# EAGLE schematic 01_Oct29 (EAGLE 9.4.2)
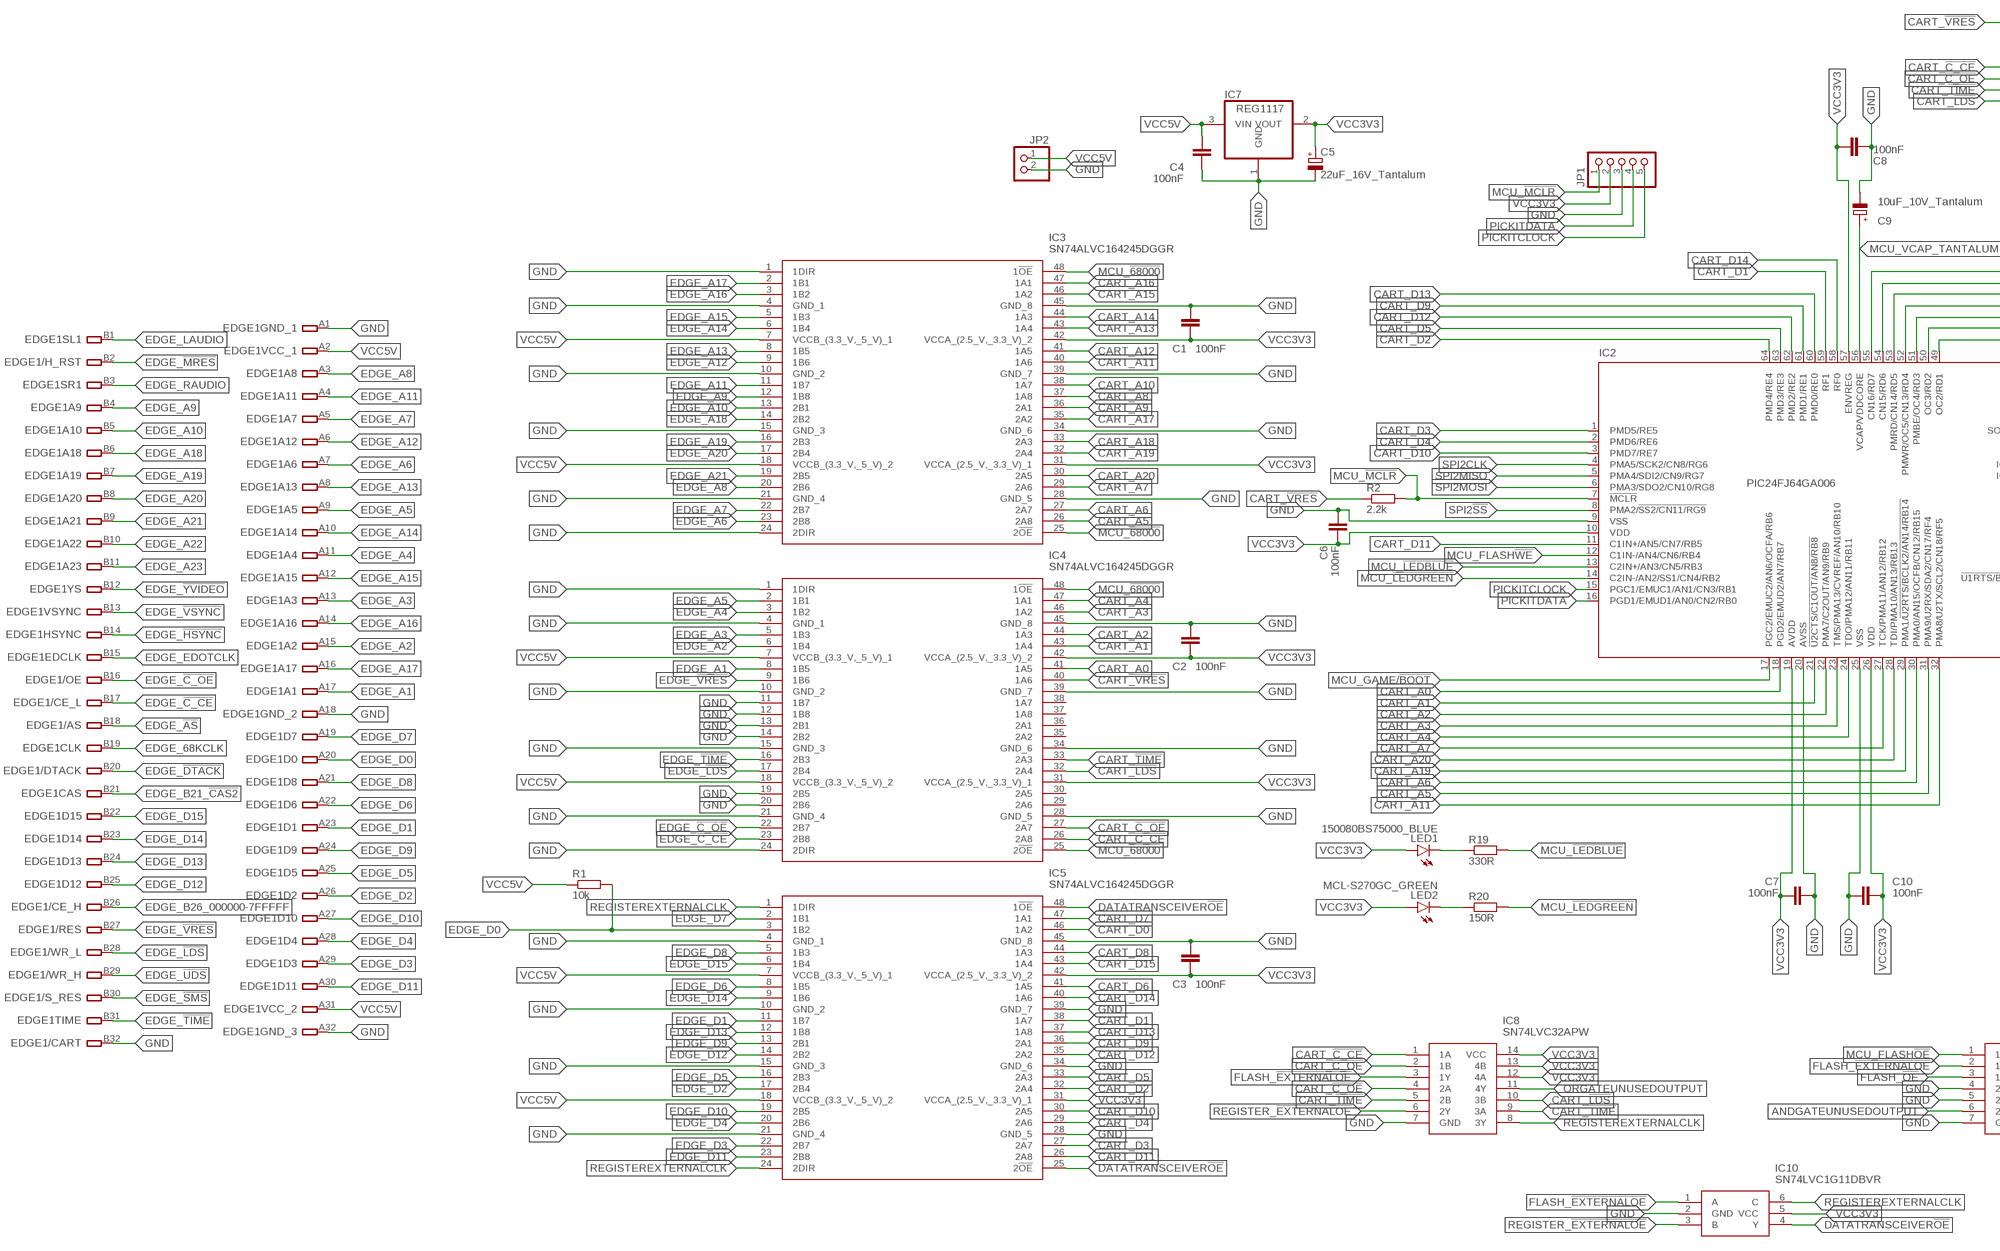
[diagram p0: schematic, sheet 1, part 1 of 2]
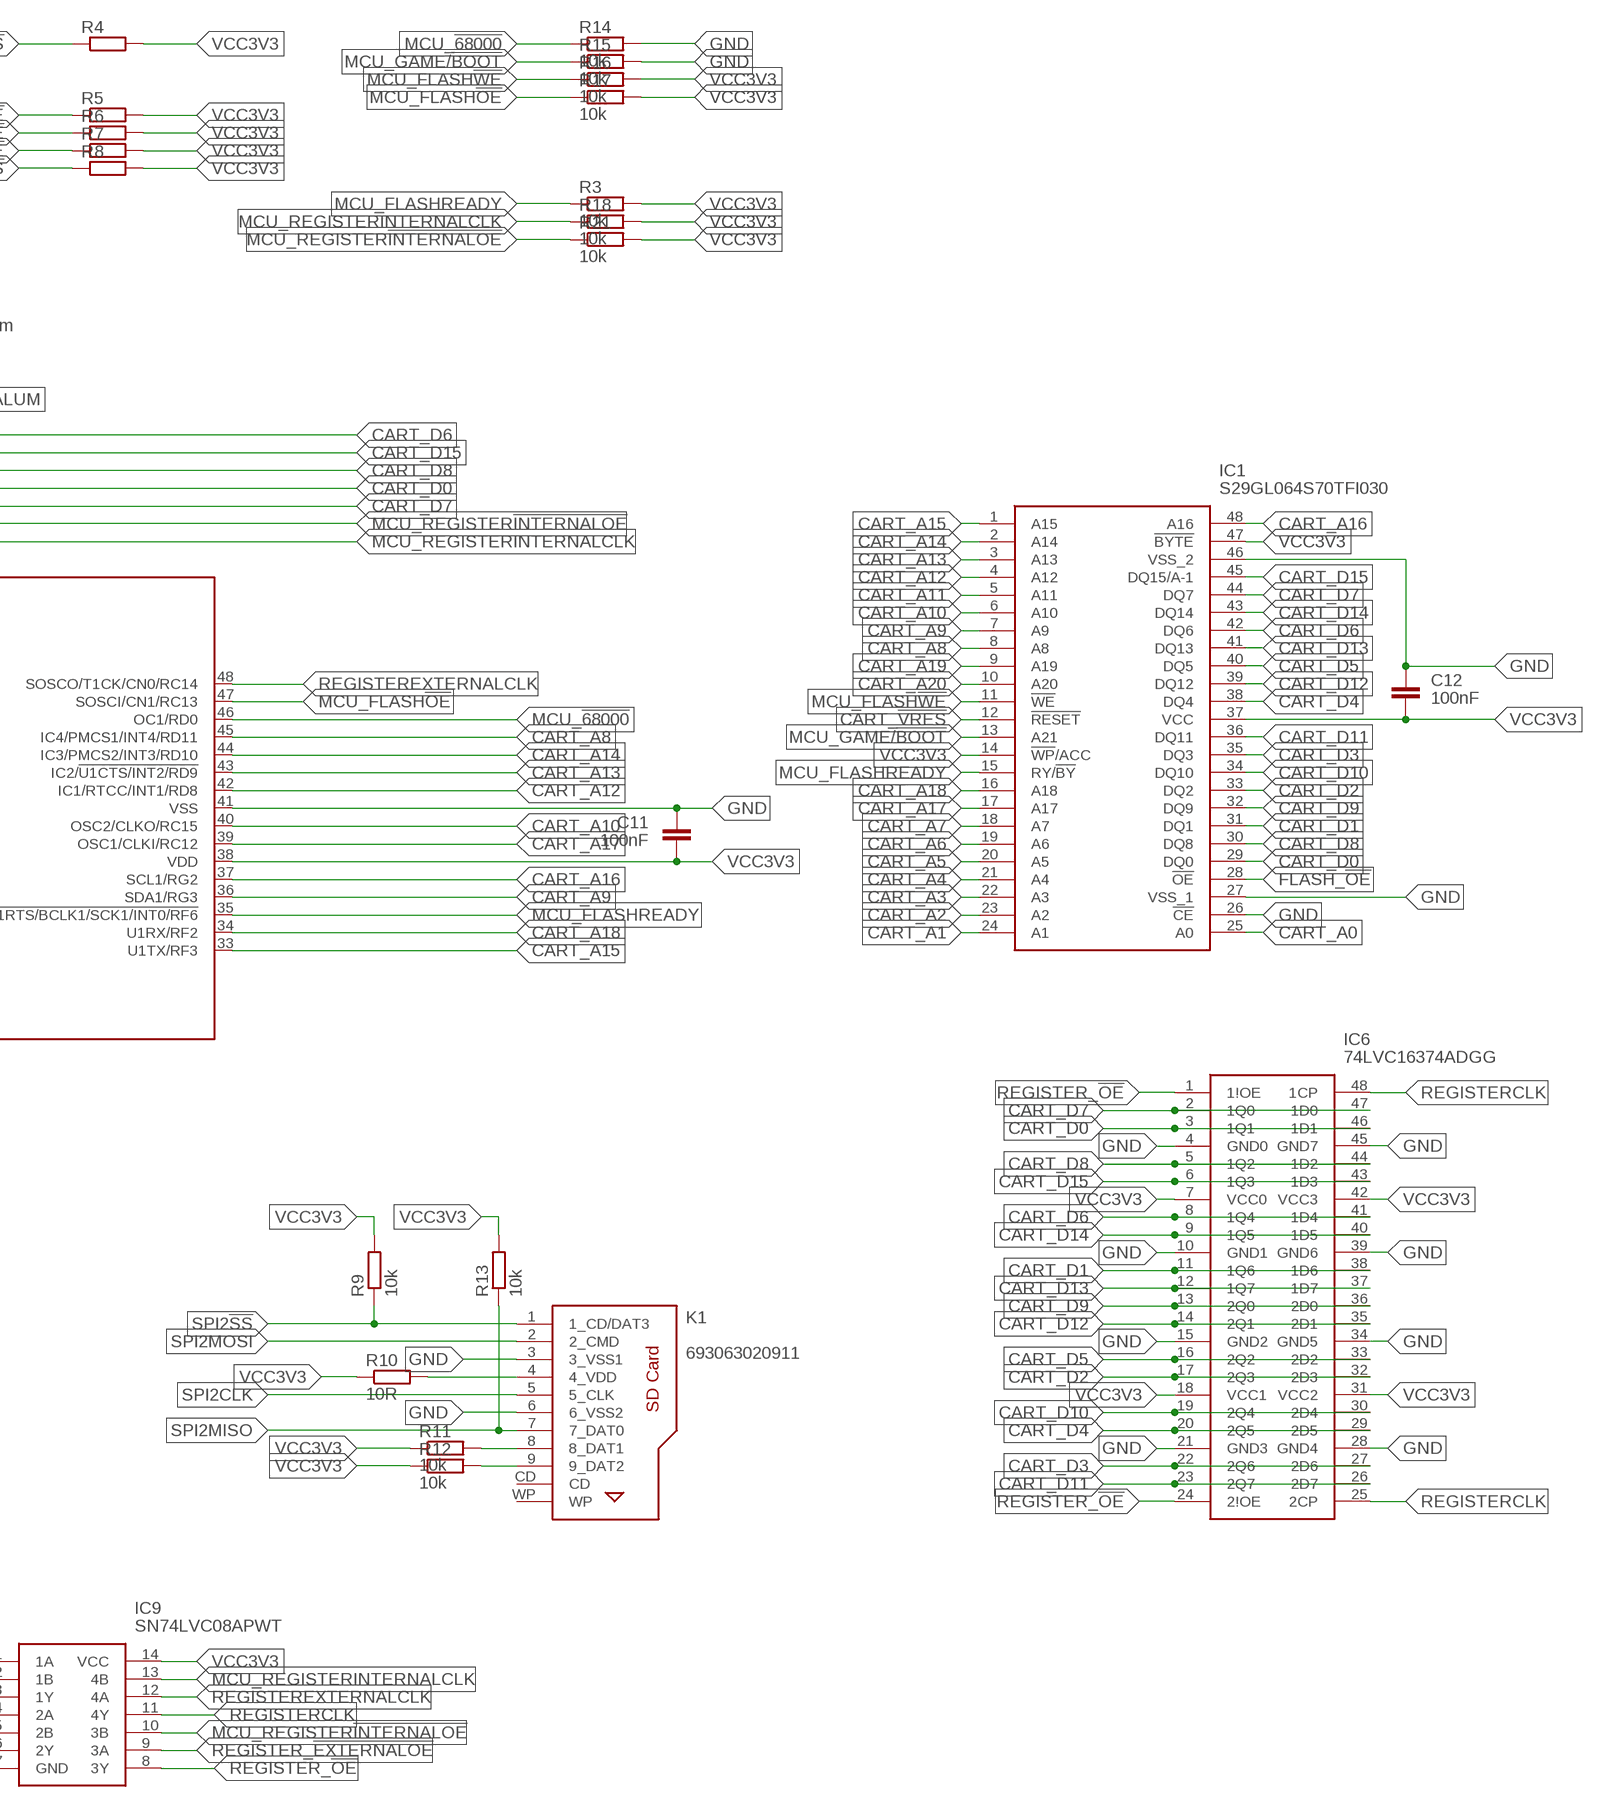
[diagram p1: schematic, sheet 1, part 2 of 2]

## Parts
C1  100nF  C-EUC0603  [C0603]
C2  100nF  C-EUC0603  [C0603]
C3  100nF  C-EUC0603  [C0603]
C4  100nF  C-EUC0603  [C0603]
C5  22uF_16V_Tantalum  CPOL-EUCT3528  [CT3528]
C6  100nF  C-EUC0603  [C0603]
C7  100nF  C-EUC0603  [C0603]
C8  100nF  C-EUC0603  [C0603]
C9  10uF_10V_Tantalum  CPOL-EUCT3216  [CT3216]
C10  100nF  C-EUC0603  [C0603]
C11  100nF  C-EUC0603  [C0603]
C12  100nF  C-EUC0603  [C0603]
EDGE1  GENESIS-LARGE  [GENESIS-LARGE]
IC1  S29GL064S70TFI030  [SOP50P2000X120-48N]
IC2  PIC24FJ64GA006  [TQFP64-10X10]
IC3  SN74ALVC164245DGGR  [SOP50P810X120-48N]
IC4  SN74ALVC164245DGGR  [SOP50P810X120-48N]
IC5  SN74ALVC164245DGGR  [SOP50P810X120-48N]
IC6  74LVC16374ADGG  [SOP50P810X120-48N]
IC7  REG1117  [SOT223]
IC8  SN74LVC32APW  [SOP65P640X120-14N]
IC9  SN74LVC08APWT  [SOP65P640X120-14N]
IC10  SN74LVC1G11DBVR  [SOT95P280X145-6N]
JP1  PINHD-1X5  [1X05]
JP2  PINHD-1X2  [1X02]
K1  693063020911  [693063020911]
LED1  150080BS75000_BLUE  LEDSML0805  [SML0805]
LED2  MCL-S270GC_GREEN  LEDSML0805  [SML0805]
R1  10k  R-EU_R0402  [R0402]
R2  2.2k  R-EU_R0402  [R0402]
R3  10k  R-EU_R0402  [R0402]
R4  10k  R-EU_R0402  [R0402]
R5  10k  R-EU_R0402  [R0402]
R6  10k  R-EU_R0402  [R0402]
R7  10k  R-EU_R0402  [R0402]
R8  10k  R-EU_R0402  [R0402]
R9  10k  R-EU_R0402  [R0402]
R10  10R  R-EU_R0402  [R0402]
R11  10k  R-EU_R0402  [R0402]
R12  10k  R-EU_R0402  [R0402]
R13  10k  R-EU_R0402  [R0402]
R14  10k  R-EU_R0402  [R0402]
R15  10k  R-EU_R0402  [R0402]
R16  10k  R-EU_R0402  [R0402]
R17  10k  R-EU_R0402  [R0402]
R18  10k  R-EU_R0402  [R0402]
R19  330R  R-EU_R0402  [R0402]
R20  150R  R-EU_R0402  [R0402]
R21  10k  R-EU_R0402  [R0402]

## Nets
ANDGATEUNUSEDOUTPUT: IC9.6(2Y)
CART_!C_CE: IC4.26(2A8) IC8.1(1A) R5.1
CART_!C_OE: IC4.27(2A7) IC8.2(1B) IC8.4(2A) R6.1
CART_!LDS: IC4.32(2A4) IC8.10(3B) R8.1
CART_!TIME: IC4.33(2A3) IC8.5(2B) IC8.9(3A) R7.1
CART_!VRES: IC1.12(!RESET) IC4.40(1A6) R2.1 R4.1
CART_A0: IC1.25(A0) IC2.18(PGD2/EMUD2/AN7/RB7) IC4.41(1A5)
CART_A1: IC1.24(A1) IC2.21(!U2CTS/C1OUT/AN8/RB8) IC4.43(1A4)
CART_A2: IC1.23(A2) IC2.22(PMA7/C2OUT/AN9/RB9) IC4.44(1A3)
CART_A3: IC1.22(A3) IC2.23(TMS/PMA13/CVREF/AN10/RB10) IC4.46(1A2)
CART_A4: IC1.21(A4) IC2.24(TDO/PMA12/AN11/RB11) IC4.47(1A1)
CART_A5: IC1.20(A5) IC2.31(PMA9/U2RX/SDA2/CN17/RF4) IC3.26(2A8)
CART_A6: IC1.19(A6) IC2.30(PMA0/AN15/OCFB/CN12/RB15) IC3.27(2A7)
CART_A7: IC1.18(A7) IC2.27(TCK/PMA11/AN12/RB12) IC3.29(2A6)
CART_A8: IC1.8(A8) IC2.45(IC4/PMCS1/INT4/RD11) IC3.37(1A8)
CART_A9: IC1.7(A9) IC2.36(SDA1/RG3) IC3.36(2A1)
CART_A10: IC1.6(A10) IC2.40(OSC2/CLKO/RC15) IC3.38(1A7)
CART_A11: IC1.5(A11) IC2.32(PMA8/U2TX/SCL2/CN18/RF5) IC3.40(1A6)
CART_A12: IC1.4(A12) IC2.42(IC1/RTCC/INT1/RD8) IC3.41(1A5)
CART_A13: IC1.3(A13) IC2.43(IC2/!U1CTS/INT2/RD9) IC3.43(1A4)
CART_A14: IC1.2(A14) IC2.44(IC3/PMCS2/INT3/RD10) IC3.44(1A3)
CART_A15: IC1.1(A15) IC2.33(U1TX/RF3) IC3.46(1A2)
CART_A16: IC1.48(A16) IC2.37(SCL1/RG2) IC3.47(1A1)
CART_A17: IC1.17(A17) IC2.39(OSC1/CLKI/RC12) IC3.35(2A2)
CART_A18: IC1.16(A18) IC2.34(U1RX/RF2) IC3.33(2A3)
CART_A19: IC1.9(A19) IC2.29(PMA1/!U2RTS/BCLK2/AN14/RB14) IC3.32(2A4)
CART_A20: IC1.10(A20) IC2.28(TDI/PMA10/AN13/RB13) IC3.30(2A5)
CART_D0: IC1.29(DQ0) IC2.52(PMWR/OC5/CN13/RD4) IC5.46(1A2) IC6.3(1Q1) IC6.46(1D1)
CART_D1: IC1.31(DQ1) IC2.59(RF1) IC5.38(1A7) IC6.11(1Q6) IC6.38(1D6)
CART_D2: IC1.33(DQ2) IC2.64(PMD4/RE4) IC5.32(2A4) IC6.17(2Q3) IC6.32(2D3)
CART_D3: IC1.35(DQ3) IC2.1(PMD5/RE5) IC5.27(2A7) IC6.22(2Q6) IC6.27(2D6)
CART_D4: IC1.38(DQ4) IC2.2(PMD6/RE6) IC5.29(2A6) IC6.20(2Q5) IC6.29(2D5)
CART_D5: IC1.40(DQ5) IC2.63(PMD3/RE3) IC5.33(2A3) IC6.16(2Q2) IC6.33(2D2)
CART_D6: IC1.42(DQ6) IC2.55(CN16/RD7) IC5.41(1A5) IC6.8(1Q4) IC6.41(1D4)
CART_D7: IC1.44(DQ7) IC2.51(PMBE/OC4/RD3) IC5.47(1A1) IC6.2(1Q0) IC6.47(1D0)
CART_D8: IC1.30(DQ8) IC2.53(PMRD/CN14/RD5) IC5.44(1A3) IC6.5(1Q2) IC6.44(1D2)
CART_D9: IC1.32(DQ9) IC2.61(PMD1/RE1) IC5.36(2A1) IC6.13(2Q0) IC6.36(2D0)
CART_D10: IC1.34(DQ10) IC2.3(PMD7/RE7) IC5.30(2A5) IC6.19(2Q4) IC6.30(2D4)
CART_D11: IC1.36(DQ11) IC2.11(C1IN+/AN5/CN7/RB5) IC5.26(2A8) IC6.23(2Q7) IC6.26(2D7)
CART_D12: IC1.39(DQ12) IC2.62(PMD2/RE2) IC5.35(2A2) IC6.14(2Q1) IC6.35(2D1)
CART_D13: IC1.41(DQ13) IC2.60(PMD0/RE0) IC5.37(1A8) IC6.12(1Q7) IC6.37(1D7)
CART_D14: IC1.43(DQ14) IC2.58(RF0) IC5.40(1A6) IC6.9(1Q5) IC6.40(1D5)
CART_D15: IC1.45(DQ15/A-1) IC2.54(CN15/RD6) IC5.43(1A4) IC6.6(1Q3) IC6.43(1D3)
DATATRANSCEIVER!OE: IC5.25(2!OE) IC5.48(1!OE) IC10.4(Y)
EDGE_68KCLK: EDGE1.B19
EDGE_!AS: EDGE1.B18
EDGE_!C_CE: EDGE1.B17 IC4.23(2B8)
EDGE_!C_OE: EDGE1.B16 IC4.22(2B7)
EDGE_!DTACK: EDGE1.B20
EDGE_!HSYNC: EDGE1.B14
EDGE_!LDS: EDGE1.B28 IC4.17(2B4)
EDGE_!MRES: EDGE1.B2
EDGE_!SMS: EDGE1.B30
EDGE_!TIME: EDGE1.B31 IC4.16(2B3)
EDGE_!UDS: EDGE1.B29
EDGE_!VRES: EDGE1.B27 IC4.9(1B6)
EDGE_!VSYNC: EDGE1.B13
EDGE_!YVIDEO: EDGE1.B12
EDGE_A1: EDGE1.A17 IC4.8(1B5)
EDGE_A2: EDGE1.A15 IC4.6(1B4)
EDGE_A3: EDGE1.A13 IC4.5(1B3)
EDGE_A4: EDGE1.A11 IC4.3(1B2)
EDGE_A5: EDGE1.A9 IC4.2(1B1)
EDGE_A6: EDGE1.A7 IC3.23(2B8)
EDGE_A7: EDGE1.A5 IC3.22(2B7)
EDGE_A8: EDGE1.A3 IC3.20(2B6)
EDGE_A9: EDGE1.B4 IC3.12(1B8)
EDGE_A10: EDGE1.B5 IC3.13(2B1)
EDGE_A11: EDGE1.A4 IC3.11(1B7)
EDGE_A12: EDGE1.A6 IC3.9(1B6)
EDGE_A13: EDGE1.A8 IC3.8(1B5)
EDGE_A14: EDGE1.A10 IC3.6(1B4)
EDGE_A15: EDGE1.A12 IC3.5(1B3)
EDGE_A16: EDGE1.A14 IC3.3(1B2)
EDGE_A17: EDGE1.A16 IC3.2(1B1)
EDGE_A18: EDGE1.B6 IC3.14(2B2)
EDGE_A19: EDGE1.B7 IC3.16(2B3)
EDGE_A20: EDGE1.B8 IC3.17(2B4)
EDGE_A21: EDGE1.B9 IC3.19(2B5)
EDGE_A22: EDGE1.B10
EDGE_A23: EDGE1.B11
EDGE_B21_!CAS2: EDGE1.B21
EDGE_B26_000000-7FFFFF: EDGE1.B26
EDGE_D0: EDGE1.A20 IC5.3(1B2) R1.2
EDGE_D1: EDGE1.A23 IC5.11(1B7)
EDGE_D2: EDGE1.A26 IC5.17(2B4)
EDGE_D3: EDGE1.A29 IC5.22(2B7)
EDGE_D4: EDGE1.A28 IC5.20(2B6)
EDGE_D5: EDGE1.A25 IC5.16(2B3)
EDGE_D6: EDGE1.A22 IC5.8(1B5)
EDGE_D7: EDGE1.A19 IC5.2(1B1)
EDGE_D8: EDGE1.A21 IC5.5(1B3)
EDGE_D9: EDGE1.A24 IC5.13(2B1)
EDGE_D10: EDGE1.A27 IC5.19(2B5)
EDGE_D11: EDGE1.A30 IC5.23(2B8)
EDGE_D12: EDGE1.B25 IC5.14(2B2)
EDGE_D13: EDGE1.B24 IC5.12(1B8)
EDGE_D14: EDGE1.B23 IC5.9(1B6)
EDGE_D15: EDGE1.B22 IC5.6(1B4)
EDGE_EDOTCLK: EDGE1.B15
EDGE_LAUDIO: EDGE1.B1
EDGE_RAUDIO: EDGE1.B3
FLASH_!EXTERNALOE: IC8.3(1Y) IC9.2(1B) IC10.1(A)
FLASH_!OE: IC1.28(!OE) IC9.3(1Y)
GND [pow]: C1.2 C2.2 C3.2 C4.1 C5.- C6.2 C7.2 C8.1 C9.- C10.1 C11.2 C12.2 EDGE1.A1 EDGE1.A18 EDGE1.A32 EDGE1.B32 IC1.26(!CE) IC1.27(VSS_1) IC1.46(VSS_2) IC2.9(VSS) IC2.20(AVSS) IC2.25(VSS) IC2.41(VSS) IC3.1(1DIR) IC3.4(GND_1) IC3.10(GND_2) IC3.15(GND_3) IC3.21(GND_4) IC3.24(2DIR) IC3.28(GND_5) IC3.34(GND_6) IC3.39(GND_7) IC3.45(GND_8) IC4.1(1DIR) IC4.4(GND_1) IC4.10(GND_2) IC4.11(1B7) IC4.12(1B8) IC4.13(2B1) IC4.14(2B2) IC4.15(GND_3) IC4.19(2B5) IC4.20(2B6) IC4.21(GND_4) IC4.24(2DIR) IC4.28(GND_5) IC4.34(GND_6) IC4.39(GND_7) IC4.45(GND_8) IC5.4(GND_1) IC5.10(GND_2) IC5.15(GND_3) IC5.21(GND_4) IC5.28(GND_5) IC5.34(GND_6) IC5.39(GND_7) IC5.45(GND_8) IC6.4(GND0) IC6.10(GND1) IC6.15(GND2) IC6.21(GND3) IC6.28(GND4) IC6.34(GND5) IC6.39(GND6) IC6.45(GND7) IC7.1(GND) IC8.7(GND) IC9.4(2A) IC9.5(2B) IC9.7(GND) IC10.2(GND) JP1.3 JP2.2 K1.3(3_VSS1) K1.6(6_VSS2) R14.2 R15.2
MCU_!68000: IC2.46(OC1/RD0) IC3.25(2!OE) IC3.48(1!OE) IC4.25(2!OE) IC4.48(1!OE) R14.1
MCU_!LEDBLUE: IC2.13(C2IN+/AN3/CN5/RB3) R19.2
MCU_!LEDGREEN: IC2.14(C2IN-/AN2/SS1/CN4/RB2) R20.2
MCU_!MCLR: IC2.7(!MCLR) JP1.1 R2.2
MCU_FLASH!OE: IC2.47(SOSCI/CN1/RC13) IC9.1(1A) R17.1
MCU_FLASH!WE: IC1.11(!WE) IC2.12(C1IN-/AN4/CN6/RB4) R16.1
MCU_FLASHREADY: IC1.15(RY/!BY) IC2.35(!U1RTS/BCLK1/SCK1/INT0/RF6) R3.1
MCU_GAME/!BOOT: IC1.13(A21) IC2.17(PGC2/EMUC2/AN6/OCFA/RB6) R15.1
MCU_REGISTER!INTERNALOE: IC2.50(OC3/RD2) IC9.10(3B) R21.1
MCU_REGISTERINTERNALCLK: IC2.49(OC2/RD1) IC9.13(4B) R18.1
MCU_VCAP_TANTALUM: C9.+ IC2.56(VCAP/VDDCORE)
N$4: LED1.C R19.1
N$5: LED2.C R20.1
ORGATEUNUSEDOUTPUT: IC8.11(4Y)
PICKITCLOCK: IC2.15(PGC1/EMUC1/AN1/CN3/RB1) JP1.5
PICKITDATA: IC2.16(PGD1/EMUD1/AN0/CN2/RB0) JP1.4
REGISTER_!EXTERNALOE: IC8.6(2Y) IC9.9(3A) IC10.3(B)
REGISTER_!OE: IC6.1(1\!OE) IC6.24(2\!OE) IC9.8(3Y)
REGISTERCLK: IC6.25(2CP) IC6.48(1CP) IC9.11(4Y)
REGISTEREXTERNALCLK: IC2.48(SOSCO/T1CK/CN0/RC14) IC5.1(1DIR) IC5.24(2DIR) IC8.8(3Y) IC9.12(4A) IC10.6(C)
SD4_VCC3V3_10R: K1.4(4_VDD) R10.2
SD8_PULLUP: K1.8(8_DAT1) R11.2
SD9_PULLUP: K1.9(9_DAT2) R12.2
SPI2!SS: IC2.8(PMA2/!SS2/CN11/RG9) K1.1(1_CD/DAT3) R9.1
SPI2CLK: IC2.4(PMA5/SCK2/CN8/RG6) K1.5(5_CLK)
SPI2MISO: IC2.5(PMA4/SDI2/CN9/RG7) K1.7(7_DAT0) R13.1
SPI2MOSI: IC2.6(PMA3/SDO2/CN10/RG8) K1.2(2_CMD)
VCC3V3: C1.1 C2.1 C3.1 C5.+ C6.1 C7.1 C8.2 C10.2 C11.1 C12.1 IC1.14(!WP!/ACC) IC1.37(VCC) IC1.47(!BYTE) IC2.10(VDD) IC2.19(AVDD) IC2.26(VDD) IC2.38(VDD) IC2.57(ENVREG) IC3.31(VCCA_(2.5_V,_3.3_V)_1) IC3.42(VCCA_(2.5_V,_3.3_V)_2) IC4.31(VCCA_(2.5_V,_3.3_V)_1) IC4.42(VCCA_(2.5_V,_3.3_V)_2) IC5.31(VCCA_(2.5_V,_3.3_V)_1) IC5.42(VCCA_(2.5_V,_3.3_V)_2) IC6.7(VCC0) IC6.18(VCC1) IC6.31(VCC2) IC6.42(VCC3) IC7.2(VOUT) IC8.12(4A) IC8.13(4B) IC8.14(VCC) IC9.14(VCC) IC10.5(VCC) JP1.2 LED1.A LED2.A R3.2 R4.2 R5.2 R6.2 R7.2 R8.2 R9.2 R10.1 R11.1 R12.1 R13.2 R16.2 R17.2 R18.2 R21.2
VCC5V: C4.2 EDGE1.A2 EDGE1.A31 IC3.7(VCCB_(3.3_V,_5_V)_1) IC3.18(VCCB_(3.3_V,_5_V)_2) IC4.7(VCCB_(3.3_V,_5_V)_1) IC4.18(VCCB_(3.3_V,_5_V)_2) IC5.7(VCCB_(3.3_V,_5_V)_1) IC5.18(VCCB_(3.3_V,_5_V)_2) IC7.3(VIN) JP2.1 R1.1
Unconnected: IC4.29(2A6) IC4.30(2A5) IC4.35(2A2) IC4.36(2A1) IC4.37(1A8) IC4.38(1A7) K1.CD K1.WP

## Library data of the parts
C1-C4 C6-C8 C10-C12 = rcl:C-EU: CAPACITOR, European symbol; SPICEPREFIX: C
C5 C9 = rcl:CPOL-EU: POLARIZED CAPACITOR, European symbol; SPICEPREFIX: C
EDGE1 = BRIANgenesis:GENESIS: Sega Genesis cartridge connector
IC1 = S29GL064S70TFI030:S29GL064S70TFI030: CYPRESS SEMICONDUCTOR - S29GL064S70TFI030 - Flash Memory, Parallel NOR, 64 Mbit, 8M x 8bit / 4M x 16bit, CFI, Parallel, TSOP, 48 Pins Source: Datasheet; DESCRIPTION: CYPRESS SEMICONDUCTOR - S29GL064S70TFI030 - Flash Memory, Parallel NOR, 64 Mbit, 8M x 8bit / 4M x 16bit, CFI, Parallel, TSOP, 48 Pins; HEIGHT: 1.2mm; MANUFACTURER_NAME: Cypress Semiconductor; MANUFACTURER_PART_NUMBER: S29GL064S70TFI030
IC2 = microchip:PIC24FJ*GA006: 64/80/100-Pin General Purpose, 16-Bit Flash Microcontrollers Source: http://ww1.microchip.com/downloads/en/DeviceDoc/39747d.pdf; MPN: PIC24FJ64GA006-I/PT; OC_FARNELL: 1146524; OC_NEWARK: 56K7343
IC3-IC5 = SN74ALVC164245DGGR:SN74ALVC164245DGGR: 16-Bit 2.5-V to 3.3-V/3.3-V To 5-V Level Shifting Transceiver With 3-State Outputs Source: Datasheet; DESCRIPTION: 16-Bit 2.5-V to 3.3-V/3.3-V To 5-V Level Shifting Transceiver With 3-State Outputs; HEIGHT: 1.2mm; MANUFACTURER_NAME: Texas Instruments; MANUFACTURER_PART_NUMBER: SN74ALVC164245DGGR; MOUSER_PART_NUMBER: 595-SNALVC164245DGGR; MOUSER_PRICE-STOCK: https://www.mouser.com/Search/Refine.aspx?Keyword=595-SNALVC164245DGGR; RS_PART_NUMBER: 3972683; RS_PRICE-STOCK: http://uk.rs-online.com/web/p/products/3972683
IC6 = 74LVC16374ADGG:74LVC16374ADGG: NXP 74LVC16374ADGG 16-Bit D Type Flip Flop IC, 3-State, 48-Pin TSSOP Source: Datasheet; DESCRIPTION: NXP 74LVC16374ADGG 16-Bit D Type Flip Flop IC, 3-State, 48-Pin TSSOP; HEIGHT: 1.2mm; MANUFACTURER_NAME: Nexperia; MANUFACTURER_PART_NUMBER: 74LVC16374ADGG
IC7 = burr-brown:REG1117: 800mA and 1A Low Dropout (LDO) Positive Regulator 1.8V, 2.5V, 2.85V, 3.3V, 5V, and Adj; MPN: REG1117; OC_FARNELL: 1097566; OC_NEWARK: 14P6981
IC8 = SN74LVC32APW:SN74LVC32APW: Quadruple 2-Input Positive-OR Gate Source: Datasheet; DESCRIPTION: Quadruple 2-Input Positive-OR Gate; HEIGHT: 1.2mm; MANUFACTURER_NAME: Texas Instruments; MANUFACTURER_PART_NUMBER: SN74LVC32APW; MOUSER_PART_NUMBER: 595-SN74LVC32APW; MOUSER_PRICE-STOCK: https://www.mouser.com/Search/Refine.aspx?Keyword=595-SN74LVC32APW; RS_PART_NUMBER: 6632874; RS_PRICE-STOCK: https://uk.rs-online.com/web/p/products/6632874
IC9 = SN74LVC08APWT:SN74LVC08APWT: Quadruple 2-Input Positive-AND Gate Source: Datasheet; DESCRIPTION: Quadruple 2-Input Positive-AND Gate; HEIGHT: 1.2mm; MANUFACTURER_NAME: Texas Instruments; MANUFACTURER_PART_NUMBER: SN74LVC08APWT
IC10 = SN74LVC1G11DBVR:SN74LVC1G11DBVR: SINGLE 3-INPUT POSITIVE-AND GATE Source: Datasheet; DESCRIPTION: SINGLE 3-INPUT POSITIVE-AND GATE; HEIGHT: 1.45mm; MANUFACTURER_NAME: Texas Instruments; MANUFACTURER_PART_NUMBER: SN74LVC1G11DBVR; MOUSER_PART_NUMBER: 595-SN74LVC1G11DBVR; MOUSER_PRICE-STOCK: https://www.mouser.com/Search/Refine.aspx?Keyword=595-SN74LVC1G11DBVR
JP1 = pinhead:PINHD-1X5: PIN HEADER
JP2 = pinhead:PINHD-1X2: PIN HEADER
K1 = SD_SHORT_Wurth_Input-Output_Connectors_rev15d:693063020911: WR-CRD SD CARD CONNECTOR PUSH & PULL SHORT TYPE WITH CARD DETECTION 9PINS=>Code : Con_I-O_COM_CRD_SD_Normal_693063020911 Details see: http://katalog.we-online.de/en/em/693_063_020_911 Created 2014-07-09, Karrer Zheng 2014 (C) Würth Elektronik
LED1 LED2 = led:LED: LED
R1-R21 = rcl:R-EU_: RESISTOR, European symbol; SPICEPREFIX: R

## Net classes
0 default: width 0.178 mm, clearance 0.178 mm
1 pow: width 0.254 mm, clearance 0.178 mm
